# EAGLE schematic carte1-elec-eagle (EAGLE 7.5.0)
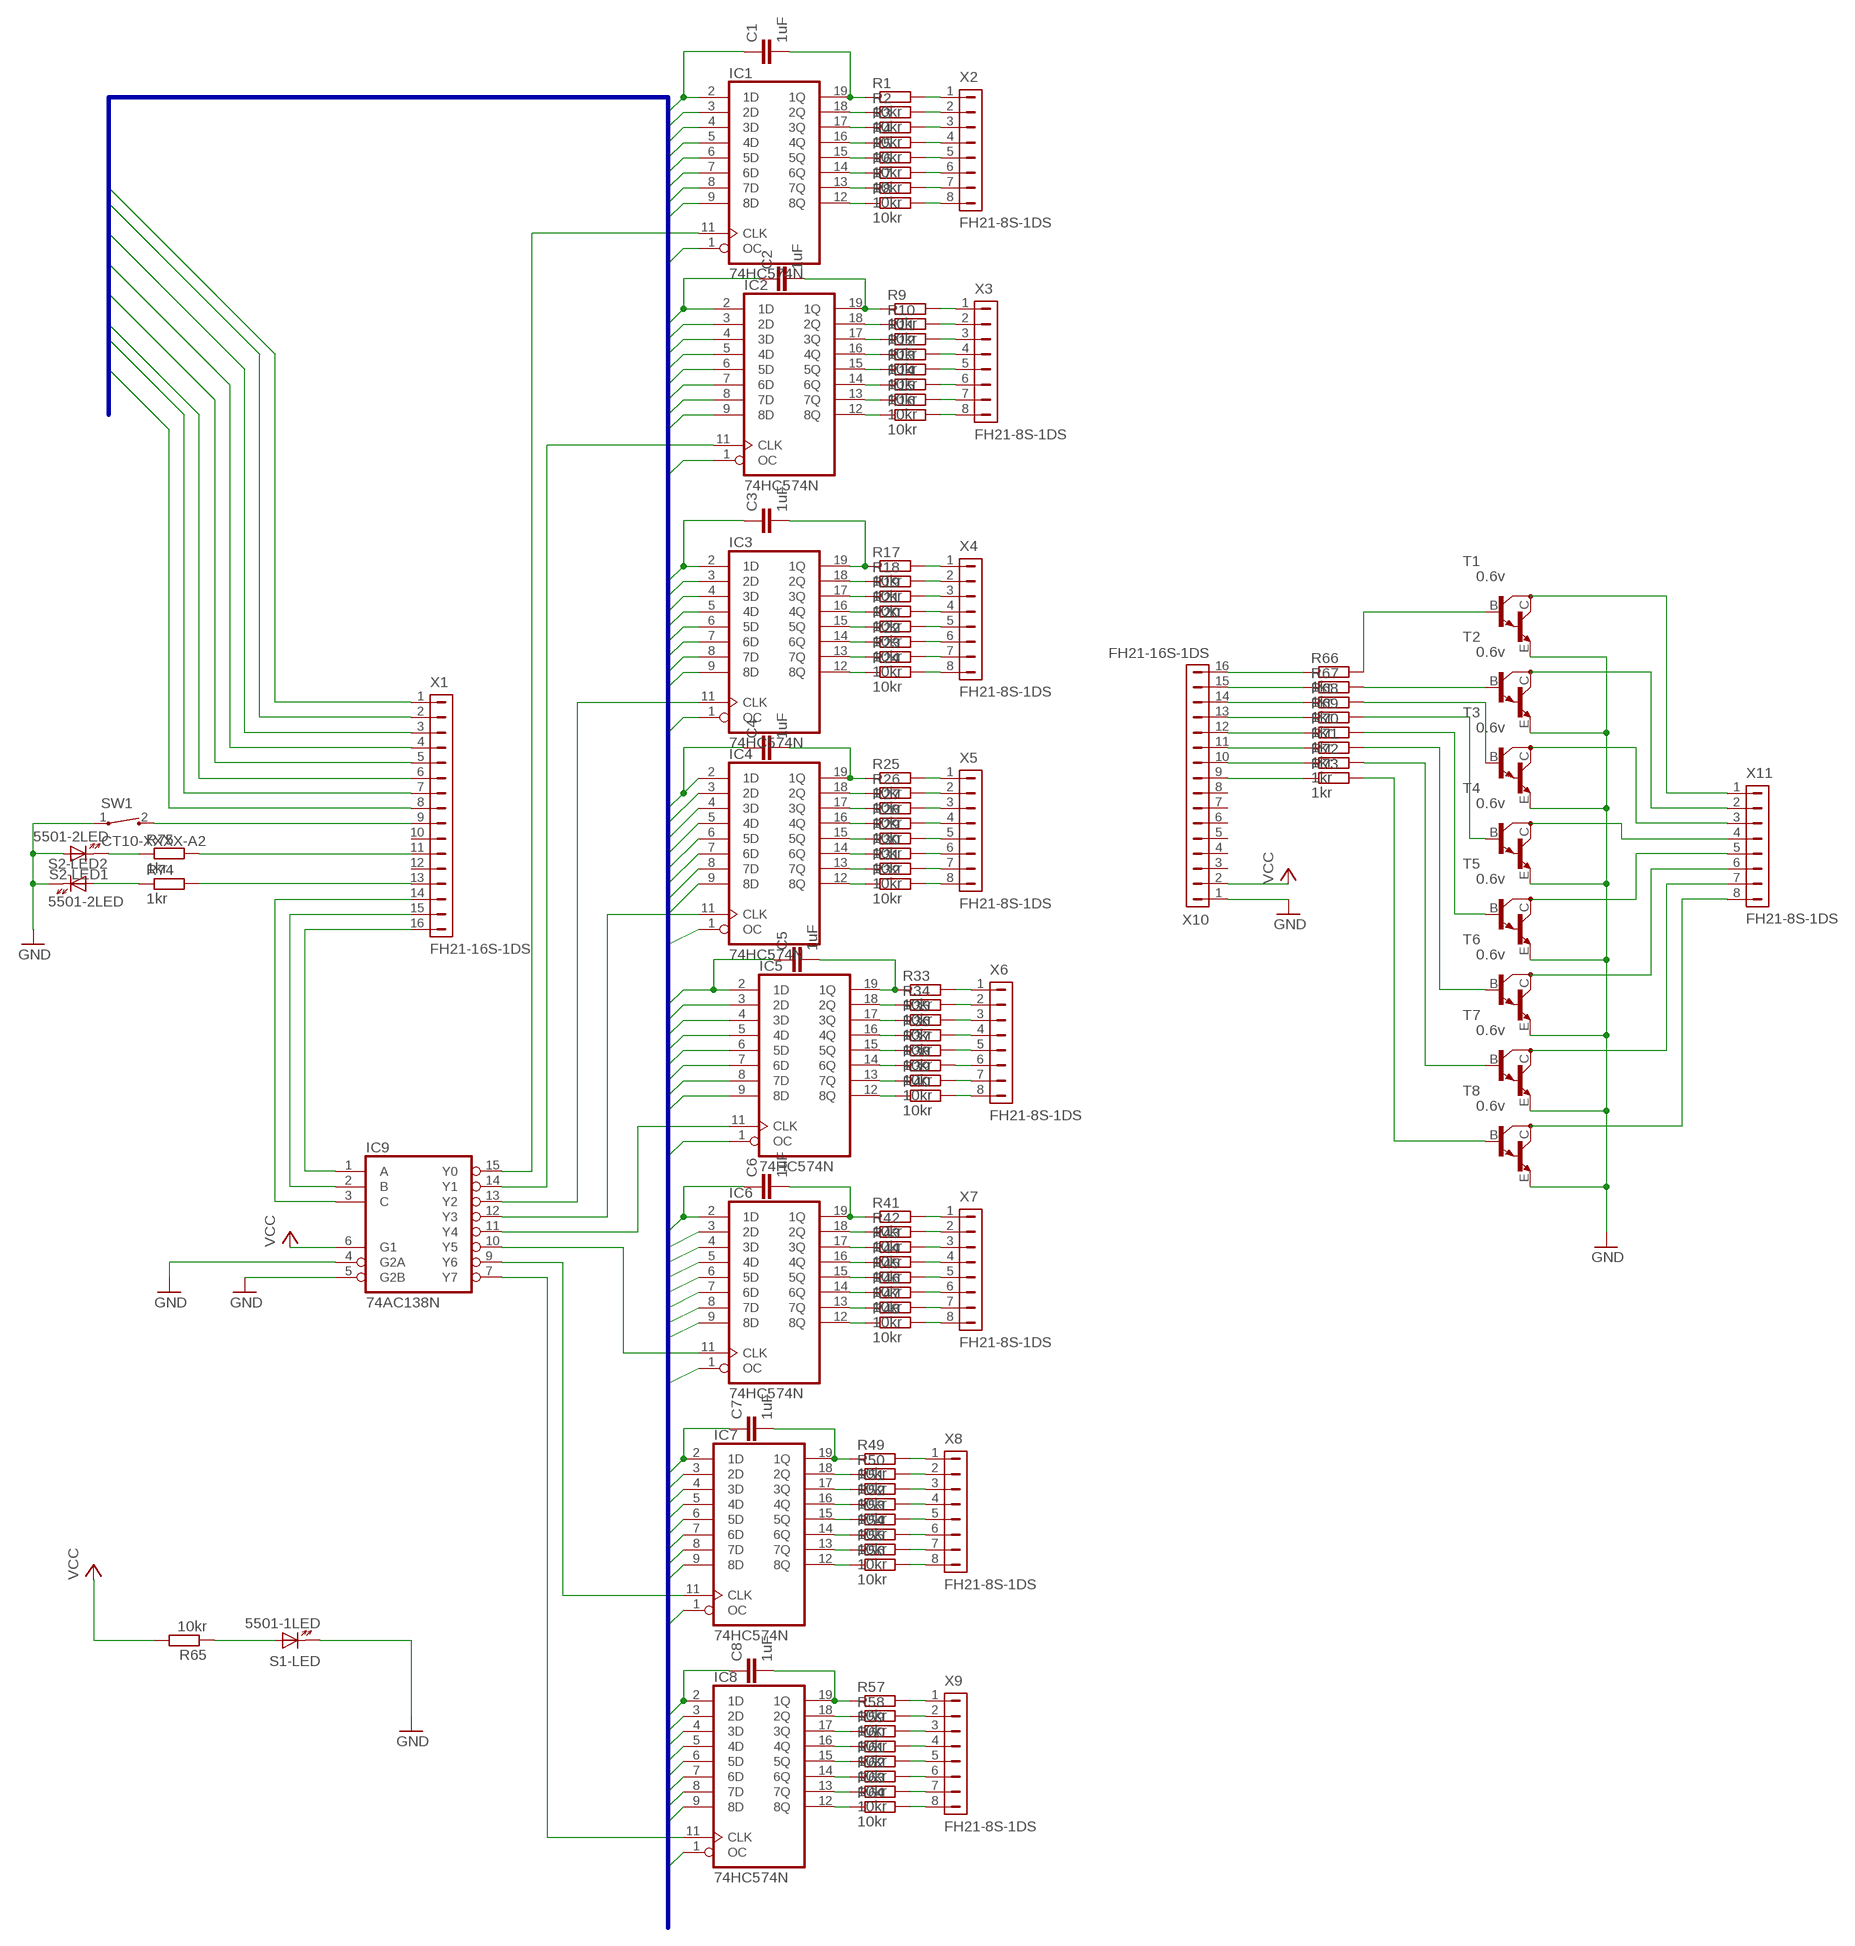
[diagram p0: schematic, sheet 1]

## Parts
C1  1uF  C-EU025-025X050  [C025-025X050]
C2  1uF  C-EU025-025X050  [C025-025X050]
C3  1uF  C-EU025-025X050  [C025-025X050]
C4  1uF  C-EU025-025X050  [C025-025X050]
C5  1uF  C-EU025-025X050  [C025-025X050]
C6  1uF  C-EU025-025X050  [C025-025X050]
C7  1uF  C-EU025-025X050  [C025-025X050]
C8  1uF  C-EU025-025X050  [C025-025X050]
IC1  74HC574N  [DIL20]
IC2  74HC574N  [DIL20]
IC3  74HC574N  [DIL20]
IC4  74HC574N  [DIL20]
IC5  74HC574N  [DIL20]
IC6  74HC574N  [DIL20]
IC7  74HC574N  [DIL20]
IC8  74HC574N  [DIL20]
IC9  74AC138N  [DIL16]
R1  10kr  R-EU_0207/10  [0207/10]
R2  10kr  R-EU_0207/10  [0207/10]
R3  10kr  R-EU_0207/10  [0207/10]
R4  10kr  R-EU_0207/10  [0207/10]
R5  10kr  R-EU_0207/10  [0207/10]
R6  10kr  R-EU_0207/10  [0207/10]
R7  10kr  R-EU_0207/10  [0207/10]
R8  10kr  R-EU_0207/10  [0207/10]
R9  10kr  R-EU_0207/10  [0207/10]
R10  10kr  R-EU_0207/10  [0207/10]
R11  10kr  R-EU_0207/10  [0207/10]
R12  10kr  R-EU_0207/10  [0207/10]
R13  10kr  R-EU_0207/10  [0207/10]
R14  10kr  R-EU_0207/10  [0207/10]
R15  10kr  R-EU_0207/10  [0207/10]
R16  10kr  R-EU_0207/10  [0207/10]
R17  10kr  R-EU_0207/10  [0207/10]
R18  10kr  R-EU_0207/10  [0207/10]
R19  10kr  R-EU_0207/10  [0207/10]
R20  10kr  R-EU_0207/10  [0207/10]
R21  10kr  R-EU_0207/10  [0207/10]
R22  10kr  R-EU_0207/10  [0207/10]
R23  10kr  R-EU_0207/10  [0207/10]
R24  10kr  R-EU_0207/10  [0207/10]
R25  10kr  R-EU_0207/10  [0207/10]
R26  10kr  R-EU_0207/10  [0207/10]
R27  10kr  R-EU_0207/10  [0207/10]
R28  10kr  R-EU_0207/10  [0207/10]
R29  10kr  R-EU_0207/10  [0207/10]
R30  10kr  R-EU_0207/10  [0207/10]
R31  10kr  R-EU_0207/10  [0207/10]
R32  10kr  R-EU_0207/10  [0207/10]
R33  10kr  R-EU_0207/10  [0207/10]
R34  10kr  R-EU_0207/10  [0207/10]
R35  10kr  R-EU_0207/10  [0207/10]
R36  10kr  R-EU_0207/10  [0207/10]
R37  10kr  R-EU_0207/10  [0207/10]
R38  10kr  R-EU_0207/10  [0207/10]
R39  10kr  R-EU_0207/10  [0207/10]
R40  10kr  R-EU_0207/10  [0207/10]
R41  10kr  R-EU_0207/10  [0207/10]
R42  10kr  R-EU_0207/10  [0207/10]
R43  10kr  R-EU_0207/10  [0207/10]
R44  10kr  R-EU_0207/10  [0207/10]
R45  10kr  R-EU_0207/10  [0207/10]
R46  10kr  R-EU_0207/10  [0207/10]
R47  10kr  R-EU_0207/10  [0207/10]
R48  10kr  R-EU_0207/10  [0207/10]
R49  10kr  R-EU_0207/10  [0207/10]
R50  10kr  R-EU_0207/10  [0207/10]
R51  10kr  R-EU_0207/10  [0207/10]
R52  10kr  R-EU_0207/10  [0207/10]
R53  10kr  R-EU_0207/10  [0207/10]
R54  10kr  R-EU_0207/10  [0207/10]
R55  10kr  R-EU_0207/10  [0207/10]
R56  10kr  R-EU_0207/10  [0207/10]
R57  10kr  R-EU_0207/10  [0207/10]
R58  10kr  R-EU_0207/10  [0207/10]
R59  10kr  R-EU_0207/10  [0207/10]
R60  10kr  R-EU_0207/10  [0207/10]
R61  10kr  R-EU_0207/10  [0207/10]
R62  10kr  R-EU_0207/10  [0207/10]
R63  10kr  R-EU_0207/10  [0207/10]
R64  10kr  R-EU_0207/10  [0207/10]
R65  10kr  R-EU_0207/10  [0207/10]
R66  1kr  R-EU_0207/5V  [0207/5V]
R67  1kr  R-EU_0207/5V  [0207/5V]
R68  1kr  R-EU_0207/5V  [0207/5V]
R69  1kr  R-EU_0207/5V  [0207/5V]
R70  1kr  R-EU_0207/5V  [0207/5V]
R71  1kr  R-EU_0207/5V  [0207/5V]
R72  1kr  R-EU_0207/5V  [0207/5V]
R73  1kr  R-EU_0207/5V  [0207/5V]
R74  1kr  R-EU_0207/10  [0207/10]
R75  1kr  R-EU_0207/10  [0207/10]
S1  5501-1LED  [5501-1LED]
S2  5501-2LED  [5501-2LED]
SW1  CT10-XXXX-A2  [CT10-XXXX-A2]
T1  0.6v  MMBTA13LT1-NPN_DARL-SOT23-BEC  [SOT23-BEC]
T2  0.6v  MMBTA13LT1-NPN_DARL-SOT23-BEC  [SOT23-BEC]
T3  0.6v  MMBTA13LT1-NPN_DARL-SOT23-BEC  [SOT23-BEC]
T4  0.6v  MMBTA13LT1-NPN_DARL-SOT23-BEC  [SOT23-BEC]
T5  0.6v  MMBTA13LT1-NPN_DARL-SOT23-BEC  [SOT23-BEC]
T6  0.6v  MMBTA13LT1-NPN_DARL-SOT23-BEC  [SOT23-BEC]
T7  0.6v  MMBTA13LT1-NPN_DARL-SOT23-BEC  [SOT23-BEC]
T8  0.6v  MMBTA13LT1-NPN_DARL-SOT23-BEC  [SOT23-BEC]
X1  FH21-16S-1DS  [FH21-16S-1DS]
X2  FH21-8S-1DS  [FH21-8S-1DS]
X3  FH21-8S-1DS  [FH21-8S-1DS]
X4  FH21-8S-1DS  [FH21-8S-1DS]
X5  FH21-8S-1DS  [FH21-8S-1DS]
X6  FH21-8S-1DS  [FH21-8S-1DS]
X7  FH21-8S-1DS  [FH21-8S-1DS]
X8  FH21-8S-1DS  [FH21-8S-1DS]
X9  FH21-8S-1DS  [FH21-8S-1DS]
X10  FH21-16S-1DS  [FH21-16S-1DS]
X11  FH21-8S-1DS  [FH21-8S-1DS]

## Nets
B$1: C1.1 C2.1 C3.1 C4.1 C5.1 C6.1 C7.1 C8.1 IC1.1(OC) IC1.2(1D) IC1.3(2D) IC1.4(3D) IC1.5(4D) IC1.6(5D) IC1.7(6D) IC1.8(7D) IC1.9(8D) IC2.1(OC) IC2.2(1D) IC2.3(2D) IC2.4(3D) IC2.5(4D) IC2.6(5D) IC2.7(6D) IC2.8(7D) IC2.9(8D) IC3.1(OC) IC3.2(1D) IC3.3(2D) IC3.4(3D) IC3.5(4D) IC3.6(5D) IC3.7(6D) IC3.8(7D) IC3.9(8D) IC4.1(OC) IC4.2(1D) IC4.3(2D) IC4.4(3D) IC4.5(4D) IC4.6(5D) IC4.7(6D) IC4.8(7D) IC4.9(8D) IC5.1(OC) IC5.2(1D) IC5.3(2D) IC5.4(3D) IC5.5(4D) IC5.6(5D) IC5.7(6D) IC5.8(7D) IC5.9(8D) IC6.1(OC) IC6.2(1D) IC6.3(2D) IC6.4(3D) IC6.5(4D) IC6.6(5D) IC6.7(6D) IC6.8(7D) IC6.9(8D) IC7.1(OC) IC7.2(1D) IC7.3(2D) IC7.4(3D) IC7.5(4D) IC7.6(5D) IC7.7(6D) IC7.8(7D) IC7.9(8D) IC8.1(OC) IC8.2(1D) IC8.3(2D) IC8.4(3D) IC8.5(4D) IC8.6(5D) IC8.7(6D) IC8.8(7D) IC8.9(8D) X1.1 X1.2 X1.3 X1.4 X1.5 X1.6 X1.7 X1.8
GND: IC9.4(G2A) IC9.5(G2B) S1.-(-LED:K) S2.+R(-LED1:A) S2.-G(-LED2:K) SW1.1 T1.E T2.E T3.E T4.E T5.E T6.E T7.E T8.E X10.1
N$1: IC6.11(CLK) IC9.10(Y5)
N$2: IC5.11(CLK) IC9.11(Y4)
N$3: IC4.11(CLK) IC9.12(Y3)
N$4: IC7.11(CLK) IC9.9(Y6)
N$5: IC8.11(CLK) IC9.7(Y7)
N$6: IC3.11(CLK) IC9.13(Y2)
N$7: IC1.11(CLK) IC9.15(Y0)
N$8: IC2.11(CLK) IC9.14(Y1)
N$9: IC9.1(A) X1.16
N$10: IC9.2(B) X1.15
N$11: IC9.3(C) X1.14
N$12: IC1.18(2Q) R2.1
N$13: R2.2 X2.2
N$14: IC1.17(3Q) R3.1
N$15: R3.2 X2.3
N$16: IC1.16(4Q) R4.1
N$17: R4.2 X2.4
N$18: IC1.15(5Q) R5.1
N$19: R66.1 X10.16
N$20: R5.2 X2.5
N$21: C1.2 IC1.19(1Q) R1.1
N$22: R1.2 X2.1
N$23: IC1.14(6Q) R6.1
N$24: R6.2 X2.6
N$25: IC1.13(7Q) R7.1
N$26: R7.2 X2.7
N$27: IC1.12(8Q) R8.1
N$28: R8.2 X2.8
N$29: C2.2 IC2.19(1Q) R9.1
N$30: R9.2 X3.1
N$31: IC2.18(2Q) R10.1
N$32: R10.2 X3.2
N$33: IC2.17(3Q) R11.1
N$34: R11.2 X3.3
N$35: IC2.16(4Q) R12.1
N$36: R12.2 X3.4
N$37: IC2.15(5Q) R13.1
N$38: R13.2 X3.5
N$39: IC2.14(6Q) R14.1
N$40: R14.2 X3.6
N$41: IC2.13(7Q) R15.1
N$42: R15.2 X3.7
N$43: IC2.12(8Q) R16.1
N$44: R16.2 X3.8
N$45: C3.2 IC3.19(1Q) R17.1
N$46: IC3.18(2Q) R18.1
N$47: IC3.17(3Q) R19.1
N$48: IC3.16(4Q) R21.1
N$49: IC3.15(5Q) R20.1
N$50: IC3.14(6Q) R22.1
N$51: IC3.13(7Q) R23.1
N$52: IC3.12(8Q) R24.1
N$53: C4.2 IC4.19(1Q) R25.1
N$54: IC4.18(2Q) R26.1
N$55: IC4.17(3Q) R27.1
N$56: IC4.16(4Q) R28.1
N$57: IC4.15(5Q) R29.1
N$58: IC4.14(6Q) R30.1
N$59: IC4.13(7Q) R31.1
N$60: IC4.12(8Q) R32.1
N$61: C5.2 IC5.19(1Q) R33.1
N$62: IC5.18(2Q) R34.1
N$63: IC5.17(3Q) R35.1
N$64: IC5.16(4Q) R36.1
N$65: IC5.15(5Q) R37.1
N$66: IC5.14(6Q) R38.1
N$67: IC5.13(7Q) R39.1
N$68: IC5.12(8Q) R40.1
N$69: C6.2 IC6.19(1Q) R41.1
N$70: IC6.18(2Q) R42.1
N$71: IC6.17(3Q) R43.1
N$72: IC6.16(4Q) R44.1
N$73: IC6.15(5Q) R45.1
N$74: IC6.14(6Q) R46.1
N$75: IC6.13(7Q) R47.1
N$76: IC6.12(8Q) R48.1
N$77: C7.2 IC7.19(1Q) R49.1
N$78: IC7.18(2Q) R50.1
N$79: IC7.17(3Q) R51.1
N$80: IC7.16(4Q) R52.1
N$81: IC7.15(5Q) R53.1
N$82: IC7.14(6Q) R54.1
N$83: IC7.13(7Q) R55.1
N$84: IC7.12(8Q) R56.1
N$85: C8.2 IC8.19(1Q) R57.1
N$86: IC8.18(2Q) R58.1
N$87: IC8.17(3Q) R59.1
N$88: IC8.16(4Q) R60.1
N$89: IC8.15(5Q) R61.1
N$90: IC8.14(6Q) R62.1
N$91: IC8.13(7Q) R63.1
N$92: IC8.12(8Q) R64.1
N$93: R17.2 X4.1
N$94: R18.2 X4.2
N$95: R19.2 X4.3
N$96: R21.2 X4.4
N$97: R20.2 X4.5
N$98: R22.2 X4.6
N$99: R23.2 X4.7
N$100: R24.2 X4.8
N$101: R25.2 X5.1
N$102: R26.2 X5.2
N$103: R27.2 X5.3
N$104: R28.2 X5.4
N$105: R29.2 X5.5
N$106: R30.2 X5.6
N$107: R31.2 X5.7
N$108: R32.2 X5.8
N$109: R33.2 X6.1
N$110: R34.2 X6.2
N$111: R35.2 X6.3
N$112: R36.2 X6.4
N$113: R37.2 X6.5
N$114: R38.2 X6.6
N$115: R39.2 X6.7
N$116: R40.2 X6.8
N$117: R41.2 X7.1
N$118: R42.2 X7.2
N$119: R43.2 X7.3
N$120: R44.2 X7.4
N$121: R45.2 X7.5
N$122: R46.2 X7.6
N$123: R47.2 X7.7
N$124: R48.2 X7.8
N$125: R49.2 X8.1
N$126: R50.2 X8.2
N$127: R51.2 X8.3
N$128: R52.2 X8.4
N$129: R53.2 X8.5
N$130: R54.2 X8.6
N$131: R55.2 X8.7
N$132: R56.2 X8.8
N$133: R57.2 X9.1
N$134: R58.2 X9.2
N$135: R59.2 X9.3
N$136: R60.2 X9.4
N$137: R61.2 X9.5
N$138: R62.2 X9.6
N$139: R63.2 X9.7
N$140: R64.2 X9.8
N$141: R67.1 X10.15
N$142: R68.1 X10.14
N$143: R69.1 X10.13
N$144: R70.1 X10.12
N$145: R71.1 X10.11
N$146: R72.1 X10.10
N$147: R73.1 X10.9
N$148: R66.2 T1.B
N$149: R69.2 T4.B
N$150: R67.2 T2.B
N$151: R68.2 T3.B
N$152: R70.2 T5.B
N$153: R71.2 T6.B
N$154: R72.2 T7.B
N$155: R73.2 T8.B
N$156: T8.C X11.8
N$157: T7.C X11.7
N$158: T6.C X11.6
N$159: T5.C X11.5
N$160: T4.C X11.4
N$161: T3.C X11.3
N$162: T2.C X11.2
N$163: T1.C X11.1
N$164: R65.1 S1.+(-LED:A)
N$165: R74.2 X1.13
N$166: R75.1 S2.-R(-LED1:K)
N$167: R75.2 X1.11
N$168: R74.1 S2.+G(-LED2:A)
N$169: SW1.2 X1.9
VCC: IC9.6(G1) R65.2 X10.2
Unconnected: S1.1A(-1:1A) S1.1B(-1:1B) S1.NC(-1:NC) S1.NO(-1:NO) S2.1A(-1:1A) S2.1B(-1:1B) S2.NC(-1:NC) S2.NO(-1:NO) X1.10 X1.12 X10.3 X10.4 X10.5 X10.6 X10.7 X10.8

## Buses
B$1

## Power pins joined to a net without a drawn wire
GND: IC1.10(GND) IC2.10(GND) IC3.10(GND) IC4.10(GND) IC5.10(GND) IC6.10(GND) IC7.10(GND) IC8.10(GND) IC9.8(GND)
VCC: IC1.20(VCC) IC2.20(VCC) IC3.20(VCC) IC4.20(VCC) IC5.20(VCC) IC6.20(VCC) IC7.20(VCC) IC8.20(VCC) IC9.16(VCC)

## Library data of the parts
C1-C8 = rcl:C-EU: CAPACITOR, European symbol
IC1-IC8 = 74xx-eu:74*574: 8-bit D type FLIP FLOP bus driver
IC9 = 74xx-eu:74*138: 3-line to 8-line DECODER/DEMULTIPLEXER
R1-R75 = resistor:R-EU_: RESISTOR, European symbol
S1 = switch:55?-1LED: PUSHBUTTON SERIES 5500 SWITCHES 1 LED Source: www.e-switch.com .. 5500.pdf
S2 = switch:55?-2LED: PUSHBUTTON SERIES 5500 SWITCHES 2 LED Source: www.e-switch.com .. 5500.pdf
SW1 = switch-coto:CT10-XXXX-: CT10 Series Molded Switch
T1-T8 = transistor:*-NPN_DARL-: NPN Darlington Transistor
X1 X10 = con-hirose:FH21-16S-1DS: FPC CONNECTOR Source: con-hirose.lbr from Bob Starr <rtzaudio@mindspring.com>; OC_FARNELL: unknown; OC_NEWARK: unknown
X2-X9 X11 = con-hirose:FH21-8S-1DS: FPC CONNECTOR Source: con-hirose.lbr from Bob Starr <rtzaudio@mindspring.com>; OC_FARNELL: unknown; OC_NEWARK: unknown

## Module ERY
Ports: 

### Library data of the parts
